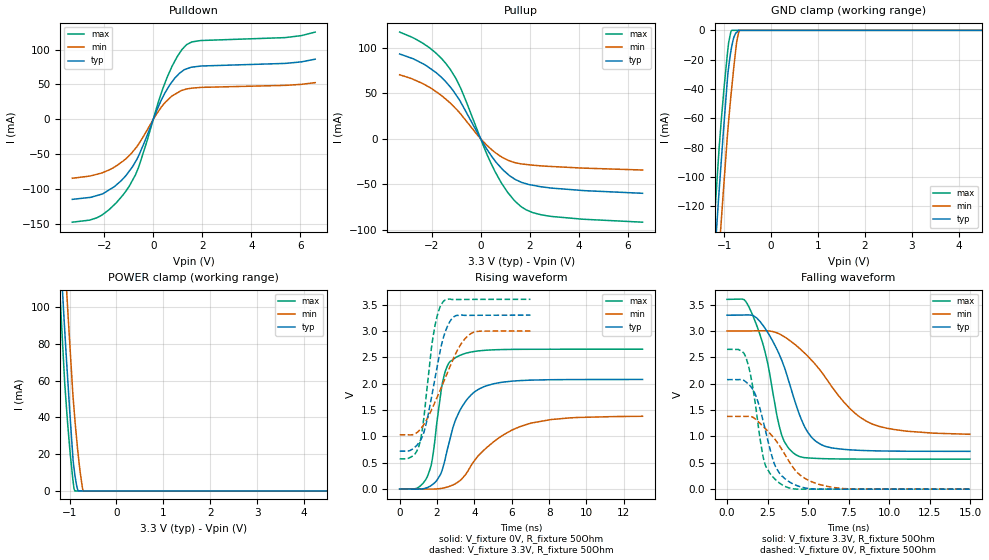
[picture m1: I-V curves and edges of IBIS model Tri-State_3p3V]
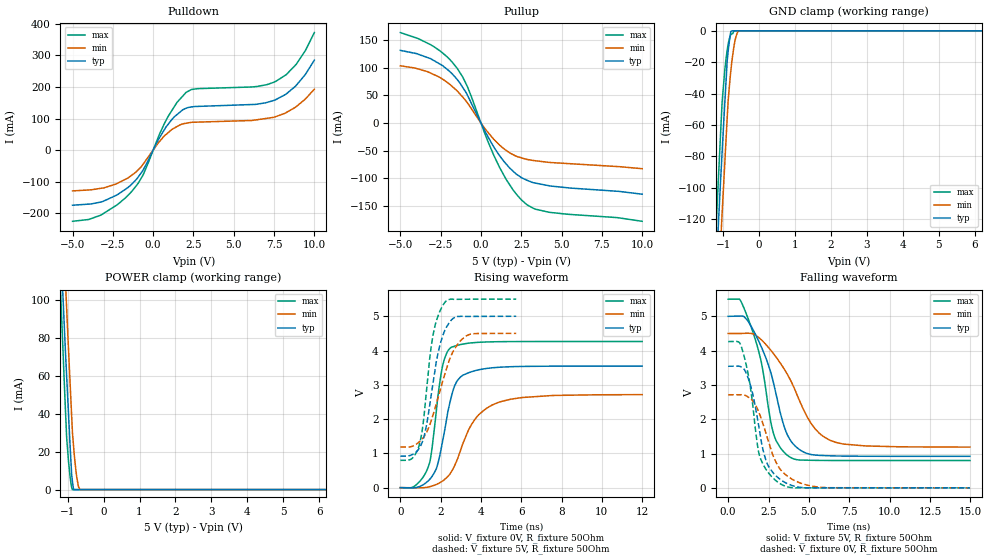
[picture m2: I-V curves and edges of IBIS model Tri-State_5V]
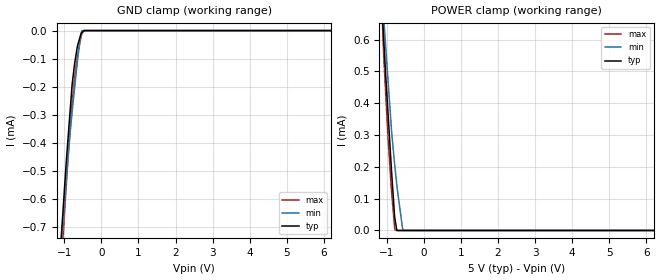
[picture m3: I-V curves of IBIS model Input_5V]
| Texas Instruments Incorporated
| 12-Bit, Dual, Ultralow Glitch, Voltage Output Digital to Analog Converter
| Marketing part#   Voltage Range   Package-type   #pins
|  DAC7552IRGTR   2.7V to 5.5V   QFN   16
|  DAC7552IRGTRG4   2.7V to 5.5V   QFN   16
|  DAC7552IRGTT   2.7V to 5.5V   QFN   16
|  DAC7552IRGTTG4   2.7V to 5.5V   QFN   16
[IBIS Ver]   3.2
[File name]   dac7552.ibs
|SIMDE Ver   V2.0 - 201002 - RHL4 - Build 372
[Date]   29 July 2010
[File Rev]   1.1
[Source]
| Texas Instruments Incorporated.
| Analog eLab Design Center, HPA
| 12500 TI Blvd
| Dallas, TX -75243
| e-Mail: elab_scm_ibis@list.ti.com
| Model generated from simulations in TISPICE
[Notes]Revision_History:
|   Rev 1.0: 07/08/2010
|   - Model generated from simulations in TISPICE
|   - Model matched to SPICE simulation
|   - Initial version of the model
|   - Model names with a trailing _3p3V stands for the Model
|   with typical voltage 3.3V - [3V,3.3V,3.6V].Model names
|   with a trailing _5V stands for the Model with typical
|   voltage 5V-[4.5V,5V,5.5V]
|   - While calculating R_pkg, L_pkg and C_pkg ignored values
|   corresponding to power and ground pins
|   - C_comp although listed in numerical order of value are
|   obtained from varying PVT conditions. For PVT conditions
|   for each specific value refer the buffer description under
|   respective [Model]. IBIS model user is responsible for using
|   appropriate C_comp to simulate for Signal Integrity
|   Rev 1.1: 07/29/2010
|   - Updated the ibis file with Vinl and Vinh values calculated
|   using VDD typ values and also added model spec
|   - Added C_comp (ON state) and C_comp (OFF state) for OUTPUT_3p3
|   and OUTPUT_5 models
|   - Removed the out of range(-VDD to 2*VDD) voltages for clamp
|   and IV curves
|   - Added Input_2v and Tri-State_2V models.
[Disclaimer]
| This model is designed as an aid for customers of Texas Instruments.
| TI and its licensors and suppliers make no warranties, either expressed
| or implied, with respect to this  model, including the warranties of
| merchantability or fitness for a particular purpose. The model is
| provided solely on an "as is" basis. The entire risk as to its quality
| and performance is with the customer.
[Copyright]
| (C) Copyright 2010 Texas Instruments Incorporated. All rights reserved.
|   COMPONENT: DAC7552
[Component]   DAC7552
[Manufacturer]  TI
[Package]  | 16 QFN - RGT package
|   typ   min   max
R_pkg   0.05563   0.05302   0.05762
L_pkg   0.90806E-09  0.85445E-09   0.94712E-09
C_pkg   0.13605E-12  0.13032E-12   0.14392E-12
|-------------------------PINS------------------------------------------------
[Pin]  signal_name model_name   R_pin   L_pin   C_pin
1   VOUTA   NC   0.05762   0.94269E-09   0.13356E-12
2   VDD   POWER   0.02709   0.65955E-09   0.17146E-12
3   GND   GND   0.02763   0.67536E-09   0.17334E-12
4   VOUTB   NC   0.05760   0.94712E-09   0.13377E-12
5   VFBB   term   0.05620   0.92447E-09   0.13070E-12
6   VREFB   NC   0.05443   0.88835E-09   0.14392E-12
7   _PD   Input   0.05302   0.86380E-09   0.14232E-12
8   DCEN   Input   0.05620   0.92447E-09   0.13060E-12
9   SDO   Tristate_output 0.05749   0.94516E-09   0.13244E-12
10   IOVDD   POWER   0.05329   0.86477E-09   0.14324E-12
11   _SYNC   Input   0.05331   0.86342E-09   0.14296E-12
12   SCLK   Input   0.05749   0.94045E-09   0.13201E-12
13   SDIN   Input   0.05620   0.91575E-09   0.13032E-12
14   _CLR   Input   0.05302   0.85445E-09   0.14200E-12
15   VREFA   NC   0.05443   0.87889E-09   0.14360E-12
16   VFBA   term   0.05620   0.91575E-09   0.13042E-12
|   Model Selectors
[Model selector] Tristate_output
Tri-State_2V   2.0V nominal tristate output
Tri-State_3p3V   3.3V nominal tristate output
Tri-State_5V   5.5V nominal tristate output
[Model selector] Input
 Input_2v   2.0V nominal input
 Input_3p3V   3.3V nominal input
 Input_5V   5V   nominal input
[Model selector] term
 term_2V   2.0V nominal termination
 term_3p3V  3.3V nominal termination
 term_5V   5V   nominal termination
|   Termination - term_3p3V
[Model] term_3p3V
Model_type Terminator
C_comp   1.0e-20F  1.0e-20F  1.0e-20F
| variable   typ   min   max
[Voltage Range]   3.30000v  3.00000V  3.60000V
[POWER Clamp Reference]  3.30000v  3.00000V  3.60000V
[GND Clamp Reference]   0.00000V  0.00000V  0.00000V
|Ambient Temperature   25   105   -40
|Junction Temperature
[Temperature Range]   25   105   -40
|   Termination - term_5V
[Model] term_5V
Model_type Terminator
C_comp   1.0e-20F  1.0e-20F  1.0e-20F
| variable   typ   min   max
[Voltage Range]   5.00000V  4.50000V  5.50000V
[POWER Clamp Reference]  5.00000V  4.50000V  5.50000V
[GND Clamp Reference]   0.00000V  0.00000V  0.00000V
|Ambient Temperature   25   105   -40
|Junction Temperature
[Temperature Range]   25   105   -40
|   Termination - term_2V
[Model] term_2V
Model_type Terminator
C_comp   1.0e-20F  1.0e-20F  1.0e-20F
| variable   typ   min   max
[Voltage Range]   2.00000v  1.80000V  2.20000V
[POWER Clamp Reference]  2.00000v  1.80000V  2.20000V
[GND Clamp Reference]   0.00000V  0.00000V  0.00000V
|Ambient Temperature   25   105   -40
|Junction Temperature
[Temperature Range]   25   105   -40
| Models and submodels in the file (9): Tri-State_3p3V (3-state), Tri-State_5V (3-state), Input_5V (Input), Input_3p3V (Input), Input_2v (Input), Tri-State_2V (3-state), term_3p3V (Terminator), term_5V (Terminator), term_2V (Terminator)
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|   Model   - Tristate_3p3V
[Model]   Tri-State_3p3V
Model_type   3-state
Polarity   Non-Inverting
Enable   Active-High
Vmeas = 1.65
Vref = 1.65
Cref = 15pF
Rref = 50
|   typ   min   max
|   (nom PVT)   (Fast PVT)   (slow PVT)
|Average
C_comp   3.626e-12   3.345e-12   3.828e-12
|ON state : BUFFER OUTPUT TURNED HIGH
|C_comp   6.462e-12   5.908e-12   6.854e-12
|OFF state: BUFFER in HIGH IMPEDANCE for IOs and 3-state,
|This is BUFFER in LOW state for OUTPUT only type
|C_comp   7.898e-13   7.811e-13   8.016e-13
| Where   nom  PVT is  Nominal Process, 3.3V, 25C
|   Fast PVT is Strong Process, 3.6V, -40C
|   Slow PVT is Weak Process, 3.0V, 105C
[Voltage Range]   3.3   3   3.6
|Ambient Temperature   25   105   -40
|Junction Temperature
[Temperature Range]   25   105   -40
[Pullup Reference]   3.3   3   3.6
[Pulldown Reference]   0   0   0
[Power Clamp Reference]   3.3   3   3.6
[GND Clamp Reference]   0   0   0
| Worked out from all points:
|   slope of the pulldown table from 0 to 0.495 V, typ, clamps not added: 12.7 ohm
|   slope of the pullup table from 0 to 0.495 V, typ, clamps not added: 23.5 ohm
|   GND clamp passes 1 mA (typ) near -0.72 V on its own axis
|   POWER clamp passes 1 mA (typ) near -0.83 V on its own axis
|   falling waveform, V_fixture 3.3V, R_fixture 50Ohm: 20-80 % time 1.85ns typ, 3.23ns min, 1.28ns max; typ from 3.3 V to 0.718 V
|   rising waveform, V_fixture 0V, R_fixture 50Ohm: 20-80 % time 1.21ns typ, 2.41ns min, 630ps max; typ from 0 V to 2.08 V
|   rising waveform, V_fixture 3.3V, R_fixture 50Ohm: 20-80 % time 857ps typ, 1.45ns min, 606ps max; typ from 0.717 V to 3.3 V
|   falling waveform, V_fixture 0V, R_fixture 50Ohm: 20-80 % time 1.11ns typ, 1.97ns min, 814ps max; typ from 2.08 V to 0 V
[Pulldown]
|   Voltage   I(typ)   I(min)   I(max)
-3.3V     -114.5mA   -84.27mA   -147.1mA
-2.094V   -107mA     -76.68mA   -137mA
-1.581V   -96.12mA   -68.21mA   -121.8mA
-985.2mV  -74.36mA   -52.04mA   -95.94mA
-571.2mV  -50.06mA   -34.05mA   -65.68mA
184.8mV   16.4mA     10.26mA    22.26mA
555.6mV   42.56mA    26.68mA    59.35mA
969.6mV   62.38mA    37.73mA    89.39mA
1.358V    72.32mA    43.49mA    106.9mA
1.942V    76.35mA    45.77mA    112.8mA
5.376V    80.1mA     48.68mA    117mA
6.6V      86.15mA    52.6mA     124.9mA
[GND Clamp]
|   Voltage   I(typ)   I(min)   I(max)
-3.3V     -1.247A    -1.267A    -1.239A
-1.218V   -161.7mA   -202.8mA   -133.7mA
-1.201V   -153.7mA   -194.9mA   -125.5mA
-1.122V   -115.5mA   -157mA     -86.73mA
-1.068V   -91.43mA   -132.2mA   -63.33mA
-924mV    -30.13mA   -68.61mA   -13.57mA
-906mV    -25.26mA   -61.87mA   -8.486mA
-841.5mV  -11.24mA   -39.7mA    0A
-792mV    -4.609mA   -24.05mA   0A
-732mV    -1.393mA   -7.54mA    0A
-669.9mV  0A         0A         0A
6.6V      0A         0A         0A
[Pullup]
|   Voltage   I(typ)   I(min)   I(max)
-3.3V     93.25mA    70.38mA    117.3mA
-2.098V   78.18mA    56.82mA    100.4mA
-1.64V    68.65mA    48.41mA    89.6mA
-1.244V   57.21mA    39.44mA    76.62mA
-805.2mV  40mA       26.93mA    55.22mA
69.3mV    -3.299mA   -2.082mA   -4.795mA
584.4mV   -24.26mA   -15.04mA   -36.01mA
1.103V    -38.93mA   -23.45mA   -59.11mA
1.625V    -47.55mA   -27.61mA   -74.19mA
2.132V    -51.28mA   -29.16mA   -81.42mA
2.899V    -54.39mA   -30.62mA   -85.62mA
6.6V      -60.1mA    -34.48mA   -91.91mA
[POWER Clamp]
|   Voltage   I(typ)   I(min)   I(max)
-3.3V     1.232A     1.247A     1.23A
-1.214V   139.3mA    178.4mA    112mA
-1.125V   97.09mA    136.7mA    69.1mA
-1.066V   71.69mA    110.6mA    45.53mA
-1.046V   63.84mA    102.1mA    38.58mA
-988.8mV  40.88mA    77.67mA    21.06mA
-924mV    16.66mA    51.02mA    5.164mA
-888mV    9.01mA     39.47mA    0A
-815.1mV  0A         19.68mA    0A
-774mV    0A         10.47mA    0A
-708mV    0A         0A         0A
6.6V      0A         0A         0A
[Ramp]
R_load = 50
|   typ   min   max
dV/dt_r   1.24689/1.20352e-09   0.827591/2.40543e-09   1.59146/6.25519e-10
dV/dt_f   1.54945/1.84518e-09   1.17556/3.22908e-09   1.81789/1.27485e-09
[Falling Waveform]
V_fixture = 3.3V
V_fixture_min = 3V
V_fixture_max = 3.6V
R_fixture = 50Ohm
C_fixture = 0F
|   Time   V(typ)   V(min)   V(max)
0s        3.3V       3V         3.6V
1.05ns    3.305V     3V         3.596V
1.525ns   3.3V       3.002V     3.341V
2.375ns   3.038V     3.003V     2.567V
3.35ns    2.464V     2.924V     1.05V
4.2ns     1.655V     2.742V     662.1mV
4.8ns     1.176V     2.577V     597.4mV
5.475ns   909.3mV    2.357V     584.1mV
8.575ns   731.6mV    1.293V     570.7mV
14.98ns   717.6mV    1.041V     570.2mV
[Rising Waveform]
V_fixture = 0V
V_fixture_min = 0V
V_fixture_max = 0V
R_fixture = 50Ohm
C_fixture = 0F
|   Time   V(typ)   V(min)   V(max)
0s        769.6pV    1.018nV    654.5pV
925ps     -4.098mV   -2.428mV   14.18mV
1.5ns     28.69mV    -3.49mV    250mV
1.75ns    80.04mV    -3.176mV   568.6mV
2.225ns   305.1mV    9.874mV    1.875V
2.4ns     513.6mV    21.88mV    2.182V
3ns       1.316V     102.6mV    2.495V
4.175ns   1.882V     615.7mV    2.619V
6.475ns   2.058V     1.187V     2.651V
13ns      2.078V     1.379V     2.652V
[Rising Waveform]
V_fixture = 3.3V
V_fixture_min = 3V
V_fixture_max = 3.6V
R_fixture = 50Ohm
C_fixture = 0F
|   Time   V(typ)   V(min)   V(max)
0s        717.4mV    1.027V     570.2mV
700ps     759.8mV    1.03V      626mV
1.05ns    886.4mV    1.111V     835.2mV
1.275ns   1.052V     1.213V     1.29V
1.8ns     1.92V      1.575V     2.915V
2.075ns   2.444V     1.798V     3.368V
2.325ns   2.852V     2.008V     3.554V
2.875ns   3.26V      2.473V     3.597V
3.85ns    3.296V     2.957V     3.599V
7ns       3.3V       3V         3.6V
[Falling Waveform]
|Gnd
V_fixture = 0V
V_fixture_min = 0V
V_fixture_max = 0V
R_fixture = 50Ohm
C_fixture = 0F
|   Time   V(typ)   V(min)   V(max)
0s        2.078V     1.38V      2.652V
1.125ns   2.045V     1.38V      2.53V
1.45ns    1.952V     1.38V      2.168V
1.725ns   1.814V     1.336V     1.661V
2.325ns   1.172V     1.16V      494.1mV
2.85ns    539.5mV    986mV      224.9mV
3.45ns    232.7mV    719.4mV    73.72mV
4.5ns     48.07mV    270.2mV    245.8uV
6.125ns   890.4uV    56.39mV    176.6uV
14.98ns   878.3nV    37.37uV    9.389nV
|   Model   - Tristate_5V
[Model]   Tri-State_5V
Model_type   3-state
Polarity   Non-Inverting
Enable   Active-High
Vmeas = 2.5
Vref = 2.5
Cref = 15pF
Rref = 50
|   typ   min   max
|   (nom PVT)   (Fast PVT)   (slow PVT)
|Average
C_comp   3.521e-12   3.462e-12   3.606e-12
|ON state : BUFFER OUTPUT TURNED HIGH
|C_comp   6.296e-12   6.474e-12   6.167e-12
|OFF state: BUFFER in HIGH IMPEDANCE for IOs and 3-state,
|This is BUFFER in LOW state for OUTPUT only type
|C_comp   7.454e-13   7.386e-13   7.563e-13
| Where   nom  PVT is  Nominal Process, 5V, 25C
|   Fast PVT is Strong Process, 5.5V, -40C
|   Slow PVT is Weak Process, 4.5V, 105C
[Voltage Range]   5   4.5   5.5
|Ambient Temperature   25   105   -40
|Junction Temperature
[Temperature Range]   25   105   -40
[Pullup Reference]   5   4.5   5.5
[Pulldown Reference]   0   0   0
[Power Clamp Reference]   5   4.5   5.5
[GND Clamp Reference]   0   0   0
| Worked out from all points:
|   slope of the pulldown table from 0 to 0.75 V, typ, clamps not added: 10.8 ohm
|   slope of the pullup table from 0 to 0.75 V, typ, clamps not added: 18.2 ohm
|   GND clamp passes 1 mA (typ) near -0.79 V on its own axis
|   POWER clamp passes 1 mA (typ) near -0.84 V on its own axis
|   falling waveform, V_fixture 5V, R_fixture 50Ohm: 20-80 % time 1.52ns typ, 2.25ns min, 1.2ns max; typ from 5 V to 0.919 V
|   rising waveform, V_fixture 0V, R_fixture 50Ohm: 20-80 % time 751ps typ, 1.37ns min, 555ps max; typ from 0 V to 3.55 V
|   rising waveform, V_fixture 5V, R_fixture 50Ohm: 20-80 % time 709ps typ, 1.04ns min, 559ps max; typ from 0.919 V to 5 V
|   falling waveform, V_fixture 0V, R_fixture 50Ohm: 20-80 % time 949ps typ, 1.3ns min, 804ps max; typ from 3.55 V to 0 V
[Pulldown]
|   Voltage   I(typ)   I(min)   I(max)
-5V       -174.5mA   -129.2mA   -225.4mA
-3.245V   -164.5mA   -121.1mA   -205.9mA
-1.321V   -107.7mA   -79.3mA    -130.5mA
-627.5mV  -63.56mA   -45.03mA   -79.14mA
800mV     73.29mA    49.58mA    94.17mA
1.479V    112.3mA    74.54mA    150.9mA
2.034V    132.4mA    84.93mA    182.2mA
2.749V    138.3mA    88.59mA    194.5mA
6.355V    144.7mA    95.39mA    201mA
7.601V    159.6mA    105.9mA    217.4mA
8.871V    204.7mA    137.5mA    271.4mA
10V       284.7mA    192.8mA    372.1mA
[GND Clamp]
|   Voltage   I(typ)   I(min)   I(max)
-5V       -2.153A    -2.159A    -2.157A
-1.195V   -150.5mA   -191.7mA   -123.6mA
-1.161V   -135.1mA   -175.4mA   -106.9mA
-1.065V   -91.8mA    -131.9mA   -61.3mA
-1.034V   -78.8mA    -118.1mA   -46.8mA
-957.5mV  -46.47mA   -84.63mA   -25.3mA
-885mV    -17.92mA   -53.37mA   -11.49mA
-805mV    -2.61mA    -29.23mA   -3.287mA
-761mV    0A         -19.71mA   -1.999mA
-657.5mV  0A         -4.753mA   0A
-561.5mV  0A         0A         0A
10V       0A         0A         0A
[Pullup]
|   Voltage   I(typ)   I(min)   I(max)
-5V       132mA      103.9mA    164.3mA
-3.125V   116.9mA    90.71mA    142.3mA
-2.151V   98.83mA    75.02mA    121.6mA
-1.496V   79.86mA    58.91mA    100.2mA
-853mV    51.37mA    37.01mA    66.89mA
423mV     -24.24mA   -16.51mA   -32.86mA
1.16V     -59.56mA   -40.22mA   -80.96mA
1.99V     -87.44mA   -57.48mA   -121.5mA
2.821V    -103.5mA   -65.98mA   -147.7mA
3.377V    -109.2mA   -68.58mA   -156.6mA
4.251V    -114.2mA   -71.62mA   -162.3mA
10V       -129.4mA   -83.02mA   -178.6mA
[POWER Clamp]
|   Voltage   I(typ)   I(min)   I(max)
-5V       2.154A     2.152A     2.166A
-1.19V    127.4mA    167mA      101.6mA
-1.107V   92.37mA    129.6mA    63.24mA
-1.06V    72.3mA     109.3mA    41.58mA
-1.029V   60.41mA    96.19mA    28.01mA
-930mV    22.55mA    55.57mA    6.453mA
-890mV    8.423mA    39.58mA    1.372mA
-869.5mV  4.767mA    31.38mA    0A
-835mV    0A         22.85mA    0A
-756.5mV  0A         8.05mA     0A
-655mV    0A         0A         0A
10V       0A         0A         0A
[Ramp]
R_load = 50
|   typ   min   max
dV/dt_r   2.12746/7.50646e-10   1.62816/1.3624e-09   2.5583/5.52871e-10
dV/dt_f   2.44885/1.52165e-09   1.98783/2.25186e-09   2.8222/1.20327e-09
[Falling Waveform]
V_fixture = 5V
V_fixture_min = 4.5V
V_fixture_max = 5.5V
R_fixture = 50Ohm
C_fixture = 0F
|   Time   V(typ)   V(min)   V(max)
0s        5V         4.5V       5.5V
775ps     5.008V     4.5V       5.454V
1.7ns     4.465V     4.451V     4.297V
2.075ns   4.088V     4.307V     3.612V
2.8ns     3.076V     3.917V     1.6V
3.375ns   1.934V     3.534V     1.086V
3.775ns   1.451V     3.217V     912.2mV
5.15ns    969.7mV    1.87V      803.1mV
6.35ns    933.3mV    1.38V      797.8mV
14.98ns   918.6mV    1.187V     796.3mV
[Rising Waveform]
V_fixture = 0V
V_fixture_min = 0V
V_fixture_max = 0V
R_fixture = 50Ohm
C_fixture = 0F
|   Time   V(typ)   V(min)   V(max)
0s        1.027nV    1.267nV    934.5pV
725ps     -3.501mV   -4.727mV   52.22mV
1.375ns   193.6mV    17.54mV    591.9mV
1.775ns   535.4mV    90.27mV    2.174V
2.075ns   1.289V     185.9mV    3.487V
2.525ns   2.639V     456.8mV    4.094V
2.85ns    3.141V     859.3mV    4.155V
3.7ns     3.412V     1.993V     4.233V
4.85ns    3.51V      2.483V     4.258V
12ns      3.546V     2.714V     4.264V
[Rising Waveform]
V_fixture = 5V
V_fixture_min = 4.5V
V_fixture_max = 5.5V
R_fixture = 50Ohm
C_fixture = 0F
|   Time   V(typ)   V(min)   V(max)
0s        918.6mV    1.186V     796.3mV
575ps     960.3mV    1.203V     849.1mV
925ps     1.137V     1.328V     1.216V
1.225ns   1.614V     1.531V     2.386V
1.6ns     2.963V     2.079V     4.372V
1.875ns   3.936V     2.629V     5.013V
2.175ns   4.543V     3.247V     5.378V
2.625ns   4.939V     3.979V     5.495V
3.3ns     4.995V     4.435V     5.497V
5.75ns    5V         4.5V       5.5V
[Falling Waveform]
|Gnd
V_fixture = 0V
V_fixture_min = 0V
V_fixture_max = 0V
R_fixture = 50Ohm
C_fixture = 0F
|   Time   V(typ)   V(min)   V(max)
0s        3.546V     2.714V     4.264V
700ps     3.544V     2.713V     4.236V
1.1ns     3.366V     2.687V     3.623V
1.525ns   2.728V     2.534V     2.405V
1.95ns    1.649V     2.146V     923.2mV
2.425ns   701mV      1.462V     484mV
3.225ns   246.1mV    542.6mV    120.4mV
4.225ns   33.03mV    187.3mV    -430.3uV
5.7ns     603.4uV    17.08mV    154.5uV
14.98ns   54.04nV    3.068uV    1.617nV
|   Model   - Input_5V
[Model]   Input_5V
Model_type   Input
Vinl = 1.5
Vinh = 3.5
|   typ   min   max
|   (nom PVT)   (Fast PVT)   (slow PVT)
|Average
C_comp   1.242e-13   1.218e-13   1.870e-13
| Where   nom  PVT is  Nominal Process, 5V   , 25C
|   Fast PVT is Strong Process,   5.5V , -40C
|   Slow PVT is Weak Process,   4.5V , 105C
[model spec]
Vinl   1.5   1.35   1.65
Vinh   3.5   3.15   3.85
[Voltage Range]   5   4.5   5.5
|Ambient Temperature   25   105   -40
|Junction Temperature
[Temperature Range]   25   105   -40
[Power Clamp Reference]   5   4.5   5.5
[GND Clamp Reference]   0   0   0
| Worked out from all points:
|   GND clamp passes 1 mA (typ) near -1.20 V on its own axis
|   POWER clamp passes 1 mA (typ) near -1.26 V on its own axis
[GND Clamp]
|   Voltage   I(typ)   I(min)   I(max)
-5V       -10.31mA   -7.971mA   -14.09mA
-1.095V   -758.5uA   -784.2uA   -881.1uA
-1.024V   -617.7uA   -662.9uA   -713.4uA
-913.5mV  -407.8uA   -476.1uA   -480.4uA
-873.5mV  -338.2uA   -408.2uA   -407.1uA
-785mV    -186.8uA   -283.3uA   -250.4uA
-720mV    -115.8uA   -200.2uA   -166.5uA
-655mV    -61.94uA   -119.3uA   -97.19uA
-576.5mV  -23.56uA   -31.37uA   -41.72uA
-523mV    -5.99uA    0A         -10.17uA
-464mV    0A         0A         0A
10V       0A         0A         0A
[POWER Clamp]
|   Voltage   I(typ)   I(min)   I(max)
-5V       10.2mA     7.871mA    13.97mA
-1.117V   673.6uA    722.7uA    646.9uA
-1.095V   623uA      685.9uA    579.1uA
-1.073V   577.2uA    649uA      524.1uA
-1.03V    487.7uA    577uA      428.2uA
-968.5mV  370uA      474uA      292.3uA
-880.5mV  201.6uA    326.6uA    134.5uA
-790mV    43.85uA    209.2uA    10.05uA
-781.5mV  36.69uA    199.8uA    2.334uA
-730mV    0A         142.5uA    0A
-563mV    0A         0A         0A
10V       0A         0A         0A
